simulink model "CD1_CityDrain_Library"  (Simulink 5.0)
settings: Solver=FixedStepDiscrete  StartTime=0  StopTime=36000  FixedStep=300  RelTol=1e-3
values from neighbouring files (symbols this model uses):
  table = A(2:end,1:end)    [CD1_mfun_rainread.m]    (also in CD1_sfun_rainread.m = [table; table(end,1)+tablestep -1])
  tablestep = tableEnd-tableStart    [CD1_sfun_flowread.m]
undefined symbols (not defined in the file or in its folder): Percent

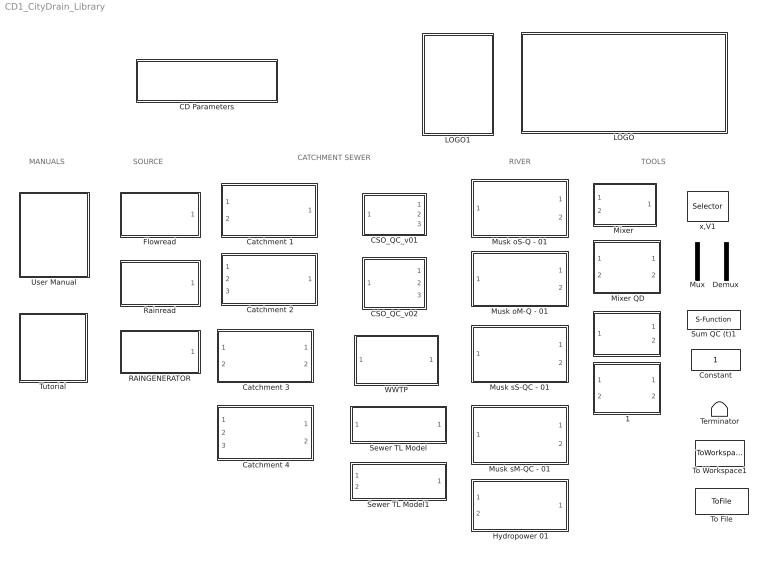
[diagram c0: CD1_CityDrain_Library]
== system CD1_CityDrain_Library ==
  note: TOOLS
  note: SOURCE
  note: RIVER
  note: CATCHMENT SEWER
  note: MANUALS
  " " : Subsystem  mask(Splitter){n_comp=1, values=40, mode=Percent [0-100]}
      mask prompts: n_comp "Number of components"; values "Fraction / Amount directed to Q1"; mode "Splitting mode"
      mask help: Splitter parameter.
      mask init:
      | % reading the toplevel systems' name 
      | % --> Plant file name;
      | tls=bdroot(gcb); 
      | % Obtaining the fixed sampling time
      | t_samp_char=get_param(tls, 'FixedStep');
      | % Convertion to numeric value
      | tstep = str2num(t_samp_char);
  " 1" : Subsystem  mask(Wrong Connect){n_comp=1, values_rain=15, mode_rain=Percent [0-100], values_dwf=23, mode_dwf=Percent [0-100]}
      mask prompts: n_comp "Number of components"; values_rain "Fraction Qr --> Qdwf"; mode_rain "Splitting mode"; values_dwf "Fraction Qdwf --> Qr"; mode_dwf "Splitting mode"
      mask help: The block simulates wrong connections given in a seperate sewer system. MAgnitudes of wrong connections are described by fraction percentages (or quanities) diverted from or to the stormwater pipe.
      mask init:
      | % reading the toplevel systems' name 
      | % --> Plant file name;
      | tls=bdroot(gcb); 
      | % Obtaining the fixed sampling time
      | t_samp_char=get_param(tls, 'FixedStep');
      | % Convertion to numeric value
      | tstep = str2num(t_samp_char);
  " Catchment 1" : Subsystem  mask(Catchment CSS - Type A){area=100, rfcoeff=0.5, initloss=1, permloss=1, n_ta=5, n_comp=1, Rain_C=[0.5], DWF_C=[1]}
      mask prompts: area "Area in [ha]"; rfcoeff "Runoff coefficient (0 - 1)"; initloss "Initial Loss in [mm]"; permloss "Permanent loss in [mm/day]"; n_ta "No of Timesteps (transport time) / No of subareas n [-]"; n_comp "No of pollutant components"; Rain_C "Vector of Rain-Conc. [g/m3]"; DWF_C "Vector of DWF-Conc. [g/m3]"
      mask help: Simple model of an urban catchment with Combined sewer system (CSS). Input ( r ) is a continuous stream of rain data in [mm/DT]. Input (dwf) is the dry weather flow in [m3/s]. Pollutants concentrations are considered as constant over time. The block contains an initial loss model for runoff generation, a time-area model for overland flow computation and a mixing model for computing runoff concentrations for n components.
      mask init:
      | % location of catchment drawing
      | x=0;
      | y=-10;
      | % reading the toplevel systems' name 
      | % --> Plant file name;
      | tls=bdroot(gcb); 
      | % Obtaining the fixed sampling time
      | t_samp_char=get_param(tls, 'FixedStep');
      | % Convertion to numeric value
      | tstep = str2num(t_samp_char); 
      | 
      | %convertion form mm/day --> mm/DT
      | permloss=permloss/86400*tstep;
      | area=area*10000;
  " Catchment 2" : Subsystem  mask(Catchment CSS - Type B){area=20, rfcoeff=0.5, initloss=1, permloss=1, n_ta=5, n_comp=1, Rain_C=[0.5]}
      mask prompts: area "Area in [ha]"; rfcoeff "Runoff coefficient (0 - 1)"; initloss "Initial Loss in [mm]"; permloss "Permanent loss in [mm/day]"; n_ta "No of Timesteps (transport time) / No of subareas n [-]"; n_comp "No of pollutant components"; Rain_C "Vector of Rain-Conc. [g/m3]"
      mask help: Simple model of an urban catchment. Input ( r ) is a continuous stream of rain data in [mm/DT]. Input (DWF) is the dry weather flow. Input (QP) is the parasite water flow entering. Pollutants concentrations for rain are considered constant over time. The block contains an initial loss model for runoff generation, a time/area model for overland flow computation and a mixing model for computing runoff concentrations for n components.
      mask init:
      | % location of catchment drawing
      | x=0;
      | y=-10;
      | % reading the toplevel systems' name 
      | % --> Plant file name;
      | tls=bdroot(gcb); 
      | % Obtaining the fixed sampling time
      | t_samp_char=get_param(tls, 'FixedStep');
      | % Convertion to numeric value
      | tstep = str2num(t_samp_char); 
      | 
      | %convertion form mm/day --> mm/DT
      | permloss=permloss/86400*tstep;
      | area=area*10000;
  " Catchment 3" : Subsystem  mask(Catchment SSS - Type A){area=20, rfcoeff=0.5, initloss=1, permloss=1, n_ta=5, n_comp=2, Rain_C=[0.5 0.2], DWF_C=[2 3]}
      mask prompts: area "Area in [ha]"; rfcoeff "Runoff coefficient (0 - 1)"; initloss "Initial Loss in [mm]"; permloss "Permanent loss in [mm/day]"; n_ta "No of Timesteps (transport time) / No of subareas n [-]"; n_comp "No of pollutant components"; Rain_C "Vector of Rain-Conc. [g/m3]"; DWF_C "Vector of DWF-Conc. [g/m3]"
      mask help: Simple model of an urban catchment with Seperate sewer system (SSS). Input ( r ) is a continuous stream of rain data in [mm/DT]. Input ( dwf ) is the dry weather flow in [m3/s]. Pollutants concentrations are considered constant over time.The block contains an initial loss model for runoff generation, a time-area model for overland flow computation and a mixing model for computing runoff concentrations for n components.
      mask init:
      | % location of catchment drawing
      | x=0;
      | y=-10;
      | % reading the toplevel systems' name 
      | % --> Plant file name;
      | tls=bdroot(gcb); 
      | % Obtaining the fixed sampling time
      | t_samp_char=get_param(tls, 'FixedStep');
      | % Convertion to numeric value
      | tstep = str2num(t_samp_char); 
      | 
      | %convertion form mm/day --> mm/DT
      | permloss=permloss/86400*tstep;
      | area=area*10000;
  " Catchment 4" : Subsystem  mask(Catchment SSS - Type B){area=20, rfcoeff=0.5, initloss=1, permloss=1, n_ta=5, n_comp=1, Rain_C=[0.5]}
      mask prompts: area "Area in [ha]"; rfcoeff "Runoff coefficient (0 - 1)"; initloss "Initial Loss in [mm]"; permloss "Permanent loss in [mm/day]"; n_ta "No of Timesteps (transport time) / No of subareas n [-]"; n_comp "No of pollutant components"; Rain_C "Vector of Rain-Conc. [g/m3]"
      mask help: Simple model of an urban catchment. Input ( r ) is a continuous stream of rain data in [mm/DT]. Input (DWF) is the dry weather flow. Input (QP) is parasite water flow entering diluting the DWF. Pollutants concentrations for stormwater Qr are considered constant over time. The block contains an initial loss model for runoff generation, a time/area model for overland flow computation and a mixing model for computing runoff concentrations for n components.
      mask init:
      | % location of catchment drawing
      | x=0;
      | y=-10;
      | % reading the toplevel systems' name 
      | % --> Plant file name;
      | tls=bdroot(gcb); 
      | % Obtaining the fixed sampling time
      | t_samp_char=get_param(tls, 'FixedStep');
      | % Convertion to numeric value
      | tstep = str2num(t_samp_char); 
      | 
      | %convertion form mm/day --> mm/DT
      | permloss=permloss/86400*tstep;
      | area=area*10000;
  " Hydropower 01" : Subsystem  mask(HYDROPOWER){n_comp=3, C_Stream=[1 2 3]}
      mask prompts: n_comp "No of components"; C_Stream "Vector of Stream-Conc. g/m3"
      mask help: Hydropower block for modelling downstream release of water. Upstream concnetration of baseflow ( qo ) and additional flow ( qa ) are considered constant. Used function: CD1_sfun_hydropower
      mask init:
      | % reading the toplevel systems' name 
      | % --> Plant file name;
      | tls=bdroot(gcb); 
      | % Obtaining the fixed sampling time
      | t_samp_char=get_param(tls, 'FixedStep');
      | % Convertion to numeric value
      | tstep = str2num(t_samp_char);
  " Mixer QD" : Subsystem  mask(Mixer QD){n_comp=3, Cmcl=[3 3 3]}
      mask prompts: n_comp "Number of pollutants [ - ]"; Cmcl "MCL - Vector of max. concentration limits [g/m3]"
      mask help: Performes mixing of pollutant fluxes Qw and Qo in accordance to their hydraulic load. Qo is considered to be the less pollluted flux. In addition the required increase of Qo is calculated for meeting required MCL (maximum concentration limits) defined by user input. Function used: CD1_sfun_mixing_QC_QD.m
      mask init:
      | % reading the toplevel systems' name 
      | % --> Plant file name;
      | tls=bdroot(gcb); 
      | % Obtaining the fixed sampling time
      | t_samp_char=get_param(tls, 'FixedStep');
      | % Convertion to numeric value
      | tstep = str2num(t_samp_char);
  CD Parameters : Subsystem  mask(City Drain 1.0 - Simulation parameters ){t_step=300, t_start=0, t_stop=36000}
      mask prompts: t_step "Sampling Time [s]"; t_start "Start Time [s]"; t_stop "Stop Time [s]"
      mask help: Block that sets the global parameters required in City Drain 1.0. Following paramters are set without user's input: - 'Solver' --> 'FixedStepDiscrete' - 'TimeSaveName' --> 'cd_time' - 'Decimation' --> '1' - 'LimitDataPoints' --> 'off'
      mask init:
      | % toplevel systems' name --> Plant file name;
      | tls=bdroot(gcb); 
      | set_param(tls, 'Solver', 'FixedStepDiscrete'); 
      | set_param(tls, 'TimeSaveName', 'cd_time');
      | set_param(tls, 'Decimation', '1');
      | set_param(tls, 'LimitDataPoints', 'off');
      | set_param(tls, 'ScreenColor', 'white');
      | 
      | tstep_char=num2str(t_step); % Setting the discrete time step
      | set_param(tls, 'FixedStep', tstep_char); 
      | 
      | tstart_char=num2str(t_start); % Setting the start time
      | set_param(tls, 'StartTime', tstart_char); 
      | 
      | tstop_char=num2str(t_stop); % Setting the stop time
      | set_param(tls, 'StopTime', tstop_char);
  CSO_QC_v01 : Subsystem  mask(CSO Typ A - Combined sewer overflow){Vmax=300, Qemax=0.1, n_comp=2}
      mask prompts: Vmax "Basin Volume [m3]"; Qemax "Maximum Effluent flow [m3/s]"; n_comp "Number of Pollutants [-]"
      mask help: Combined sewer overflow structure. Diverts the inflow given into effluent and overflow. The model implemented consideres hydraulics and pollutant routing by full mixing in the structure. Function used: CD1_sfun_cso_A.m
      mask init:
      | % reading the toplevel systems' name 
      | % --> Plant file name;
      | tls=bdroot(gcb); 
      | % Obtaining the fixed sampling time
      | t_samp_char=get_param(tls, 'FixedStep');
      | % Convertion to numeric value
      | tstep = str2num(t_samp_char);
  CSO_QC_v02 : Subsystem  mask(CSO Typ B - Combined sewer overflow){Vmax=300, Qemax=0.1, n_comp=1, n_sed=[0.2]}
      mask prompts: Vmax "Basin Volume (m3)"; Qemax "Maximum Effluent flow [m3/s]"; n_comp "Number of Pollutants [-]"; n_sed "n-sed (Vect. of Sed. Coefficients)"
      mask help: Combined sewer overflow structure. Diverts the inflow given into effluent and overflow. The model implemented consideres hydraulics and pollutant routing by full mixing in the structure. In addition to Type A a retenetion/sedimentation factor is introduced. The factor may be used for applying different ratios in pollutant concentration for effluent flow (QE) and overflow (QW). Function used: CD1_sfun_cso_B.m
      mask init:
      | % reading the toplevel systems' name 
      | % --> Plant file name;
      | tls=bdroot(gcb); 
      | % Obtaining the fixed sampling time
      | t_samp_char=get_param(tls, 'FixedStep');
      | % Convertion to numeric value
      | tstep = str2num(t_samp_char);
  Constant : Constant
  Demux : Demux  Outputs=[13,1]
  Flowread : Subsystem  mask(CD1_Flowread){table0='Input_CSO_QC_Test_01.txt', dtype=Composite sample, crep=off}
      mask prompts: table0 "Filename"; dtype "Data type"; crep "Cylic repitition"
      mask help: Reads flowdata (Q) and substance concentration (Ci) associated from ascii file. Used function: CD1_sfun_flowread.m CD1_mfun_flowread.m
      mask init:
      | table=CD1_mfun_flowread(table0);
      | 
      | 
      | % reading the toplevel systems' name 
      | % --> Plant file name;
      | tls=bdroot(gcb); 
      | % Obtaining the fixed sampling time
      | t_samp_char=get_param(tls, 'FixedStep');
      | % Convertion to numeric value
      | tstep = str2num(t_samp_char);
  LOGO : Subsystem
  LOGO1 : Subsystem
  "Mixer " : Subsystem  mask(Mixer){n_comp=1}
      mask prompts: n_comp "Number of pollutants [ - ]"
      mask help: Performes mixing of pollutant fluxes Q1 and Q2 in accordance to their hydraulic load. Function used: CD1_sfun_mixing_QC.m
      mask init:
      | % reading the toplevel systems' name 
      | % --> Plant file name;
      | tls=bdroot(gcb); 
      | % Obtaining the fixed sampling time
      | t_samp_char=get_param(tls, 'FixedStep');
      | % Convertion to numeric value
      | tstep = str2num(t_samp_char);
  Musk oM-Q - 01 : Subsystem  mask(Muskingum - Cunge flood rooting (original scheme)){K=900, X=0.2, N=2}
      mask prompts: K "K (travel time of one subreach) [ s ]"; X "X (weighing factor) [ - ]"; N "N (Number of sub-reaches) [ - ]"
      mask help: Flood routing using the original scheme by Muskingum-Cunge for multiple river stretches for hydraulic routing only. The block accepts flow inputs and returns effluent fluxes and current stated of retained volume. Intial Conditions: V=0; and Qe=0; Function used: CD1_sfun_Muskingum_oM_Q.m
      mask init:
      | m=[5,5];%Offset for arrow 
      | l=[65,15];%Offset for arrow 
      | x=0; 
      | y=-15; %Offset for river
      | 
      | % reading the toplevel systems' name-> Plant file name;
      | tls=bdroot(gcb); 
      | % Obtaining the fixed sampling time
      | tstep_char=get_param(tls, 'FixedStep');
      | % Convertion to numeric value
      | dt = str2num(tstep_char); 
      | 
      | 
      | 
      | %Muskingum parameters
      | D=K.*(1-X)+0.5.*dt;
      | C0=(0.5.*dt-K.*X)./D;
      | C1=(0.5.*dt+K.*X)./D;
      | C2=(K.*(1-X)-0.5.*dt)./D;
  Musk oS-Q - 01 : Subsystem  mask(Muskingum - Cunge flood rooting (original scheme)){K=300, X=0.2}
      mask prompts: K "K (travel time of the reach) [s]"; X "X (weighing factor)  [ - ]"
      mask help: Flood routing unsing the original scheme by Muskingum-Cunge for a single river stretch for hydraulic routing only. The block accepts flow inputs and returns effluent fluxes and current stated of retained volume. Intial Conditions: V=0; and Qe=0; Function used: CD1_sfun_Muskingum_oS_Q.m
      mask init:
      | % reading the toplevel systems' name 
      | % --> Plant file name;
      | tls=bdroot(gcb); 
      | % Obtaining the fixed sampling time
      | t_samp_char=get_param(tls, 'FixedStep');
      | % Convertion to numeric value
      | dt = str2num(t_samp_char); 
      | 
      | %Muskingum parameters
      | D=K.*(1-X)+0.5.*dt;
      | C0=(0.5.*dt-K.*X)./D;
      | C1=(0.5.*dt+K.*X)./D;
      | C2=(K.*(1-X)-0.5.*dt)./D;
  Musk sM-QC - 01 : Subsystem  mask(Muskingum - Cunge flood rooting - simplified scheme){K=300, X=0.3, n_comp=1, N=1}
      mask prompts: K "K (travel time of a subreach) [s]"; X "X (weighing factor)  [ - ]"; n_comp "Number of pollutants [ - ]"; N "N (Number of sub-reaches) [ - ]"
      mask help: Flood routing using the Muskingum-Cunge scheme for multiple river stretches for hydraulic and pollutant routing. The block accepts flow inputs and returns effluent fluxes and current stated of retained volume. Intial Conditions: V=0; and Qe=0; Function used: CD1_sfun_Muskingum_sM_QC.m
      mask init:
      | m=[5,5];%Offset for arrow 
      | l=[65,15];%Offset for arrow 
      | x=0; 
      | y=-15; %Offset for river
      | 
      | % reading the toplevel systems' name 
      | % --> Plant file name;
      | tls=bdroot(gcb); 
      | % Obtaining the fixed sampling time
      | t_samp_char=get_param(tls, 'FixedStep');
      | % Convertion to numeric value
      | dt = str2num(t_samp_char); 
      | 
      | %Muskingum parameters
      | CA=0.5.*dt-K.*X;
      | CB=0.5.*dt+K.*(1-X);
  Musk sS-QC - 01 : Subsystem  mask(Muskingum - Cunge flood rooting ){K=300, X=0.2, n_comp=1}
      mask prompts: K "K (travel time of the reach) [s]"; X "X (weighing factor)  [ - ]"; n_comp "Number of pollutants n [ - ]"
      mask help: Flood routing using the Muskingum-Cunge scheme for a single river stretch. Routing is provide for hydraulics and pollutants using a simplified discrete scheme. The block accepts flow inputs and returns effluent fluxes and current states of retained volume. Intial Conditions: V=0; and Qe=0; Function used: CD1_sfun_Muskingum_sS_QC.m
      mask init:
      | % reading the toplevel systems' name 
      | % --> Plant file name;
      | tls=bdroot(gcb); 
      | % Obtaining the fixed sampling time
      | t_samp_char=get_param(tls, 'FixedStep');
      | % Convertion to numeric value
      | dt = str2num(t_samp_char); 
      | 
      | %Muskingum parameters
      | CA=0.5.*dt-K.*X;
      | CB=0.5.*dt+K.*(1-X);
  Mux : Mux  Inputs=[13,1]
  RAINGENERATOR : Subsystem  mask(Rain Generator){param=[1,3,0.2,0.3]}
      mask prompts: param "Parameters [a,b,c,d]"
      mask help: Generates rain pattern by means of stochstics.
      mask init:
      | a=param(1);
      | b=param(2);
      | c=param(3);
      | d=param(4);
      | 
      | % reading the toplevel systems' name 
      | % --> Plant file name;
      | tls=bdroot(gcb); 
      | % Obtaining the fixed sampling time
      | t_samp_char=get_param(tls, 'FixedStep');
      | % Convertion to numeric value
      | t_step = str2num(t_samp_char);
  Rainread : Subsystem  mask(Rain Read){table0='test2.km2', crep=off}
      mask prompts: table0 "Filename"; crep "Cylic repitition"
      mask help: Read raindata from ASCII File in following formats: *.ixx ... Format used by the Austrian Hydrographic Service. *.km2 ... Format used in the Mouse Software from DHI (Danish Hydraulic Institute) *.mse ... modified mse format used in Mouse Software from DHI (Danish Hydraulic Institute) Used function: CD1_mfun_rainread.m
      mask init:
      | % cache table size set to 1000
      | %table=zeros(1000,2)
      | [table,tablestep]=CD1_mfun_rainread(table0);
      | 
      | % reading the toplevel systems' name 
      | % --> Plant file name;
      | tls=bdroot(gcb); 
      | % Obtaining the fixed sampling time
      | t_samp_char=get_param(tls, 'FixedStep');
      | % Convertion to numeric value
      | tstep = str2num(t_samp_char);
  Sewer TL Model : Subsystem  mask(SEWER Translation Model){n_elem=5, n_comp=1}
      mask prompts: n_elem "Transport time in No of Timesteps ()"; n_comp "Number of Components ()"
      mask help: Block accepts Qi as inflow carrying a number of pollutants (n_comp) Output is the flow at the end of sewer Qe Function used: CD1_sfun_sewer_tlmodel.m
      mask init:
      | %arrow location in icon
      | kx=70;
      | ky=25;
      | % picture location
      | x=20;y=25;
      | 
      | 
      | % reading the toplevel systems' name 
      | % --> Plant file name;
      | tls=bdroot(gcb); 
      | % Obtaining the fixed sampling time
      | t_samp_char=get_param(tls, 'FixedStep');
      | % Convertion to numeric value
      | tstep = str2num(t_samp_char);
  Sewer TL Model1 : Subsystem  mask(SEWER TL - Translation Model){n_elem=5, n_comp=1}
      mask prompts: n_elem "Transport time in No of Timesteps ()"; n_comp "Number of Components ()"
      mask help: Block accepts Qi as inflow carrying a number of pollutants (n_comp). Flow of parasite water (Qp) is optional. Output is the flow at the end of sewer Qe. Function used: CD1_sfun_sewer_tlmodel.m
      mask init:
      | %arrow location in icon
      | kx=70;
      | ky=25;
      | % picture location
      | x=20;y=25;
      | 
      | 
      | % reading the toplevel systems' name 
      | % --> Plant file name;
      | tls=bdroot(gcb); 
      | % Obtaining the fixed sampling time
      | t_samp_char=get_param(tls, 'FixedStep');
      | % Convertion to numeric value
      | tstep = str2num(t_samp_char);
  Sum QC (t)1 : S-Function  FunctionName=CD1_sfun_sum_QC  Parameters=n_p, tstep  mask(Cumulation of Masses){n_p=1}
      mask prompts: n_p "Number of pollutants [ - ]"
      mask help: This block returns the total hydraulic load V [m3] and the pollutant load M [g] during the simulation run. Function used: CD1_sfun_sum_QC_t.m
      mask init:
      | % reading the toplevel systems' name 
      | % --> Plant file name;
      | tls=bdroot(gcb); 
      | % Obtaining the fixed sampling time
      | t_samp_char=get_param(tls, 'FixedStep');
      | % Convertion to numeric value
      | tstep = str2num(t_samp_char);
  Terminator : Terminator
  To File : ToFile  Filename=output.mat
  To Workspace1 : ToWorkspace  VariableName=yout  SampleTime=-1  SaveFormat=Array
  Tutorial : Subsystem
  User Manual : Subsystem
  WWTP : Subsystem  mask(WWTP){REmin=[0.85 0.8 0.75], Cemax=[5 .2 .5], n_comp=3}
      mask prompts: REmin "Removal Efficiency REmin [-]"; Cemax "Maximum effluent concnetration Cemax [g/m³]"; n_comp "Number of Components ()"
      mask help: Simple WWTP model. Inflow given is treated according to userdefined maximum concnetration limits and treatment efficiencies. Function used: CD1_sfun_WWTP.m
      mask init:
      | % reading the toplevel systems' name 
      | % --> Plant file name;
      | tls=bdroot(gcb); 
      | % Obtaining the fixed sampling time
      | t_samp_char=get_param(tls, 'FixedStep');
      | % Convertion to numeric value
      | tstep = str2num(t_samp_char); 
      | 
      | RE=REmin;
      | for i=1:n_comp
      | 	if REmin(i) < 0 
      | 		RE(i)=0;
      | 		fprintf('WARNING, Block WWTP:  Removal efficientc of component %u has set to 0, User input REmin <0 \n',i);
      | 	elseif REmin(i) > 1
      | 		RE(i)=1;
      | 		fprintf('WARNING, Block WWTP:  Removal efficientc of component %u has set to 1, User input REmin >1 \n',i);
      | 	else
      | 		RE(i)=REmin(i);
      | 	end
      | end
      | fprintf('\n');
  x,V1 : Selector  Elements=(1:14)  InputPortWidth=3*14

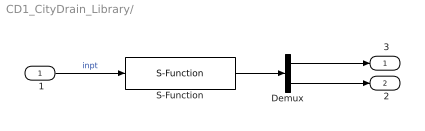
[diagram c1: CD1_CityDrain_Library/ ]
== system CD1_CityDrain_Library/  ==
  " 1" : Inport
  Demux : Demux  Outputs=2
  S-Function : S-Function  FunctionName=CD1_sfun_splitter  Parameters=n_comp,values,mode,tstep
  " 3" : Outport
  " 2" : Outport  Port=2
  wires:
  " 1"/1 -> S-Function/1  "inpt"
  S-Function/1 -> Demux/1
  Demux/1 -> " 3"/1
  Demux/2 -> " 2"/1

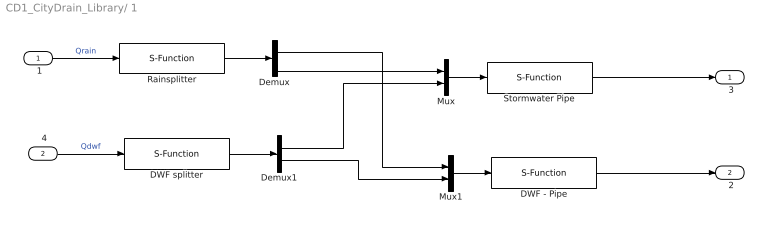
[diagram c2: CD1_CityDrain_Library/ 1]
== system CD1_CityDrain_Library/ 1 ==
  " 1" : Inport
  " 4" : Inport  Port=2
  DWF - Pipe : S-Function  FunctionName=CD1_sfun_mixing_QC  Parameters=n_comp,tstep
  DWF splitter : S-Function  FunctionName=CD1_sfun_splitter  Parameters=n_comp,values_dwf,mode_dwf,tstep
  Demux : Demux  Outputs=2
  Demux1 : Demux  Outputs=2
  Mux : Mux  Inputs=2
  Mux1 : Mux  Inputs=2
  Rainsplitter : S-Function  FunctionName=CD1_sfun_splitter  Parameters=n_comp,values_rain,mode_rain,tstep
  Stormwater Pipe : S-Function  FunctionName=CD1_sfun_mixing_QC  Parameters=n_comp,tstep
  " 3" : Outport
  " 2" : Outport  Port=2
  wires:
  " 1"/1 -> Rainsplitter/1  "Qrain"
  Rainsplitter/1 -> Demux/1
  " 4"/1 -> DWF splitter/1  "Qdwf"
  DWF splitter/1 -> Demux1/1
  Mux/1 -> Stormwater Pipe/1
  Demux/2 -> Mux/1
  Demux1/1 -> Mux/2
  Mux1/1 -> DWF - Pipe/1
  Demux/1 -> Mux1/1
  Demux1/2 -> Mux1/2
  DWF - Pipe/1 -> " 2"/1
  Stormwater Pipe/1 -> " 3"/1

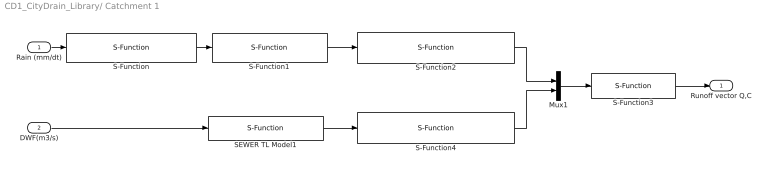
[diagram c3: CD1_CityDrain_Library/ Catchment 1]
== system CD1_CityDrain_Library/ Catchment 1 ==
  Rain (mm/dt) : Inport
  DWF(m3/s) : Inport  Port=2
  Mux1 : Mux  Inputs=[n_comp+1,n_comp+1]
  S-Function : S-Function  FunctionName=CD1_sfun_catchment_lossmodel  Parameters=initloss,permloss,rfcoeff
  S-Function1 : S-Function  FunctionName=CD1_sfun_catchment_tamodel  Parameters=n_ta
  S-Function2 : S-Function  FunctionName=CD1_sfun_catchment_flowmodel_SW  Parameters=area,n_comp,Rain_C,tstep
  S-Function3 : S-Function  FunctionName=CD1_sfun_mixing_QC  Parameters=n_comp,tstep
  S-Function4 : S-Function  FunctionName=CD1_sfun_catchment_flowmodel_DWF  Parameters=n_comp,DWF_C,tstep
  SEWER TL Model1 : S-Function  FunctionName=CD1_sfun_sewer_tlmodel  Parameters=n_ta,0,tstep
  Runoff vector Q,C : Outport
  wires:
  S-Function/1 -> S-Function1/1
  Rain (mm/dt)/1 -> S-Function/1
  DWF(m3/s)/1 -> SEWER TL Model1/1
  Mux1/1 -> S-Function3/1
  S-Function3/1 -> Runoff vector Q,C/1
  S-Function1/1 -> S-Function2/1
  SEWER TL Model1/1 -> S-Function4/1
  S-Function2/1 -> Mux1/1
  S-Function4/1 -> Mux1/2

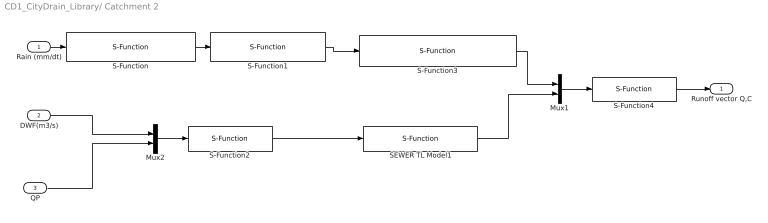
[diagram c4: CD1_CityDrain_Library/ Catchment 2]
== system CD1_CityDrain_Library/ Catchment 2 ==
  Rain (mm/dt) : Inport
  DWF(m3/s) : Inport  Port=2
  QP : Inport  Port=3
  Mux1 : Mux  Inputs=[n_comp+1,n_comp+1]
  Mux2 : Mux  Inputs=[n_comp+1,n_comp+1]
  S-Function : S-Function  FunctionName=CD1_sfun_catchment_lossmodel  Parameters=initloss,permloss,rfcoeff
  S-Function1 : S-Function  FunctionName=CD1_sfun_catchment_tamodel  Parameters=n_ta
  S-Function2 : S-Function  FunctionName=CD1_sfun_mixing_QC  Parameters=n_comp,tstep
  S-Function3 : S-Function  FunctionName=CD1_sfun_catchment_flowmodel_SW  Parameters=area,n_comp,Rain_C,tstep
  S-Function4 : S-Function  FunctionName=CD1_sfun_mixing_QC  Parameters=n_comp,tstep
  SEWER TL Model1 : S-Function  FunctionName=CD1_sfun_sewer_tlmodel  Parameters=n_ta,n_comp,tstep
  Runoff vector Q,C : Outport
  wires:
  S-Function/1 -> S-Function1/1
  Rain (mm/dt)/1 -> S-Function/1
  Mux1/1 -> S-Function4/1
  S-Function4/1 -> Runoff vector Q,C/1
  S-Function3/1 -> Mux1/1
  S-Function1/1 -> S-Function3/1
  Mux2/1 -> S-Function2/1
  S-Function2/1 -> SEWER TL Model1/1
  DWF(m3/s)/1 -> Mux2/1
  QP/1 -> Mux2/2
  SEWER TL Model1/1 -> Mux1/2

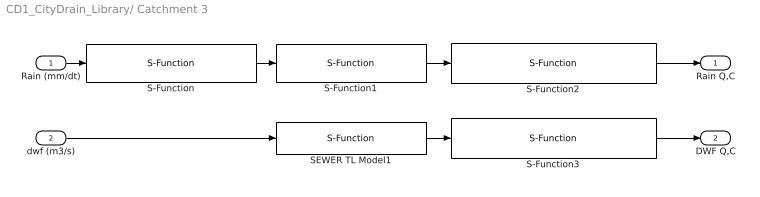
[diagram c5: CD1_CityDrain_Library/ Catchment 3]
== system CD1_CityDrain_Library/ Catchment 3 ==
  Rain (mm/dt) : Inport
  dwf (m3/s) : Inport  Port=2
  S-Function : S-Function  FunctionName=CD1_sfun_catchment_lossmodel  Parameters=initloss,permloss,rfcoeff
  S-Function1 : S-Function  FunctionName=CD1_sfun_catchment_tamodel  Parameters=n_ta
  S-Function2 : S-Function  FunctionName=CD1_sfun_catchment_flowmodel_SW  Parameters=area,n_comp,Rain_C,tstep
  S-Function3 : S-Function  FunctionName=CD1_sfun_catchment_flowmodel_DWF  Parameters=n_comp,DWF_C,tstep
  SEWER TL Model1 : S-Function  FunctionName=CD1_sfun_sewer_tlmodel  Parameters=n_ta,0,tstep
  Rain Q,C : Outport
  DWF Q,C : Outport  Port=2
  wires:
  S-Function2/1 -> Rain Q,C/1
  S-Function/1 -> S-Function1/1
  Rain (mm/dt)/1 -> S-Function/1
  dwf (m3/s)/1 -> SEWER TL Model1/1
  S-Function1/1 -> S-Function2/1
  SEWER TL Model1/1 -> S-Function3/1
  S-Function3/1 -> DWF Q,C/1

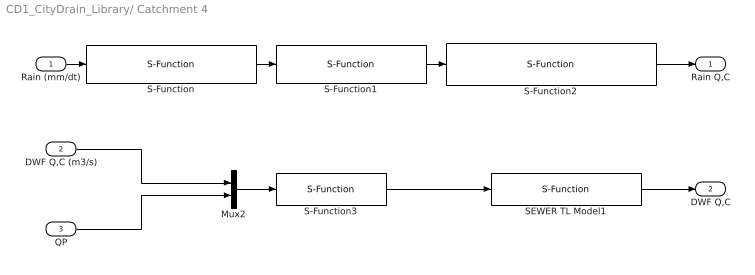
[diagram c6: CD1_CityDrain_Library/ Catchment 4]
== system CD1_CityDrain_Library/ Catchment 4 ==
  Rain (mm/dt) : Inport
  DWF Q,C (m3/s) : Inport  Port=2
  QP : Inport  Port=3
  Mux2 : Mux  Inputs=[n_comp+1,n_comp+1]
  S-Function : S-Function  FunctionName=CD1_sfun_catchment_lossmodel  Parameters=initloss,permloss,rfcoeff
  S-Function1 : S-Function  FunctionName=CD1_sfun_catchment_tamodel  Parameters=n_ta
  S-Function2 : S-Function  FunctionName=CD1_sfun_catchment_flowmodel_SW  Parameters=area,n_comp,Rain_C,tstep
  S-Function3 : S-Function  FunctionName=CD1_sfun_mixing_QC  Parameters=n_comp,tstep
  SEWER TL Model1 : S-Function  FunctionName=CD1_sfun_sewer_tlmodel  Parameters=n_ta,n_comp,tstep
  Rain Q,C : Outport
  DWF Q,C : Outport  Port=2
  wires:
  S-Function2/1 -> Rain Q,C/1
  S-Function/1 -> S-Function1/1
  Rain (mm/dt)/1 -> S-Function/1
  S-Function1/1 -> S-Function2/1
  SEWER TL Model1/1 -> DWF Q,C/1
  Mux2/1 -> S-Function3/1
  S-Function3/1 -> SEWER TL Model1/1
  DWF Q,C (m3/s)/1 -> Mux2/1
  QP/1 -> Mux2/2

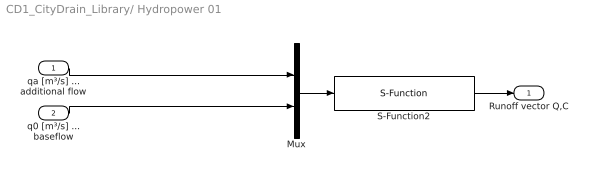
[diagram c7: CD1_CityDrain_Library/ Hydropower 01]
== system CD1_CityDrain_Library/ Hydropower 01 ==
  qa [m³/s] ... additional flow : Inport
  q0 [m³/s] ... baseflow : Inport  Port=2
  Mux : Mux  Inputs=2
  S-Function2 : S-Function  FunctionName=CD1_sfun_hydropower  Parameters=n_comp,C_Stream,tstep
  Runoff vector Q,C : Outport
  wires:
  Mux/1 -> S-Function2/1
  S-Function2/1 -> Runoff vector Q,C/1
  q0 [m³/s] ... baseflow/1 -> Mux/2
  qa [m³/s] ... additional flow/1 -> Mux/1

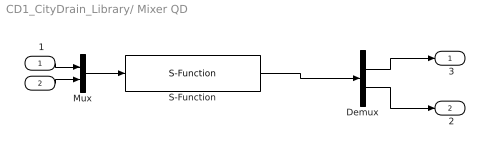
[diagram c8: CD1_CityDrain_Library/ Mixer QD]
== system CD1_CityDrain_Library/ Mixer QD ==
  " 1" : Inport
  " " : Inport  Port=2
  Demux : Demux  Outputs=[ (n_comp+1) (n_comp+1)]
  Mux : Mux  Inputs=2
  S-Function : S-Function  FunctionName=CD1_sfun_mixing_QC_QD  Parameters=n_comp,tstep,Cmcl
  " 3" : Outport
  " 2" : Outport  Port=2
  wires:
  " "/1 -> Mux/2
  " 1"/1 -> Mux/1
  Mux/1 -> S-Function/1
  Demux/1 -> " 3"/1
  Demux/2 -> " 2"/1
  S-Function/1 -> Demux/1

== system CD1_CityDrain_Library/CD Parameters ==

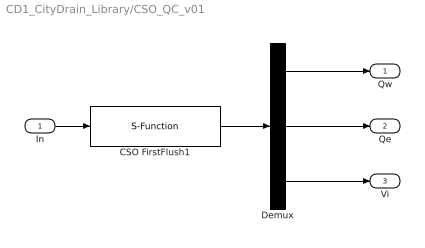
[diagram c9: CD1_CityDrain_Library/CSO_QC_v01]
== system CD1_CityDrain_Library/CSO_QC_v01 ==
  In : Inport
  CSO FirstFlush1 : S-Function  FunctionName=CD1_sfun_cso_A  Parameters=Vmax,Qemax,n_comp,tstep
  Demux : Demux  Outputs=[ (n_comp+1) (n_comp+1) (n_comp+1)]
  Qw : Outport
  Qe : Outport  Port=2
  Vi : Outport  Port=3
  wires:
  In/1 -> CSO FirstFlush1/1
  CSO FirstFlush1/1 -> Demux/1
  Demux/1 -> Qw/1
  Demux/2 -> Qe/1
  Demux/3 -> Vi/1

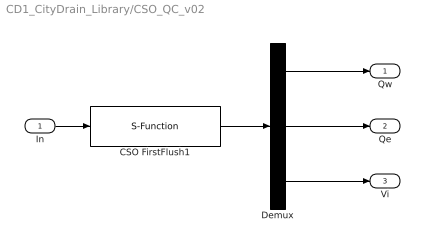
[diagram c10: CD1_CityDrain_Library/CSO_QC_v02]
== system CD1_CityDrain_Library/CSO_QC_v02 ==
  In : Inport
  CSO FirstFlush1 : S-Function  FunctionName=CD1_sfun_cso_B  Parameters=Vmax,Qemax,n_comp,n_sed,tstep
  Demux : Demux  Outputs=[ (n_comp+1) (n_comp+1) (n_comp+1)]
  Qw : Outport
  Qe : Outport  Port=2
  Vi : Outport  Port=3
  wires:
  In/1 -> CSO FirstFlush1/1
  CSO FirstFlush1/1 -> Demux/1
  Demux/1 -> Qw/1
  Demux/2 -> Qe/1
  Demux/3 -> Vi/1

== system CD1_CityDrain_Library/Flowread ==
  flowread : S-Function  FunctionName=CD1_sfun_flowread  Parameters=dtype,crep,table,tstep
  out_1 : Outport
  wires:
  flowread/1 -> out_1/1

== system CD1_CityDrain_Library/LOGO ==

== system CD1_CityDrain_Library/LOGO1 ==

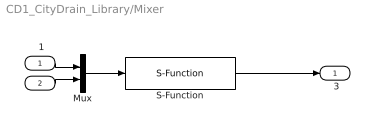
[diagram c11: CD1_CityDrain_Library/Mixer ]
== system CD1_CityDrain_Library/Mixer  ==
  " 1" : Inport
  " " : Inport  Port=2
  Mux : Mux  Inputs=[n_comp+1,n_comp+1]
  S-Function : S-Function  FunctionName=CD1_sfun_mixing_QC  Parameters=n_comp,tstep
  " 3" : Outport
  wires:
  " "/1 -> Mux/2
  S-Function/1 -> " 3"/1
  " 1"/1 -> Mux/1
  Mux/1 -> S-Function/1

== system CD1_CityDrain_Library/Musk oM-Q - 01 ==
  Qi : Inport
  Demux : Demux  Outputs=[N+1,N]
  S-Function1 : S-Function  FunctionName=CD1_sfun_Muskingum_oM_Q  Parameters=dt,N,K,X,C0,C1,C2
  Q : Outport
  V : Outport  Port=2
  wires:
  Qi/1 -> S-Function1/1
  Demux/2 -> V/1
  Demux/1 -> Q/1
  S-Function1/1 -> Demux/1

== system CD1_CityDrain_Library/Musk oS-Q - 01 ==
  Qi : Inport
  Demux : Demux  Outputs=2
  S-Function1 : S-Function  FunctionName=CD1_sfun_Muskingum_oS_Q  Parameters=dt, K, X, C0, C1, C2
  Qe : Outport
  V : Outport  Port=2
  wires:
  S-Function1/1 -> Demux/1
  Demux/1 -> Qe/1
  Demux/2 -> V/1
  Qi/1 -> S-Function1/1

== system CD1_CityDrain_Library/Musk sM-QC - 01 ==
  Qi : Inport
  Demux : Demux  Outputs=2
  S-Function1 : S-Function  FunctionName=CD1_sfun_Muskingum_sM_QC  Parameters=dt, K, X, CA, CB, n_comp,N
  Qe : Outport
  V : Outport  Port=2
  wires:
  S-Function1/1 -> Demux/1
  Demux/1 -> Qe/1
  Demux/2 -> V/1
  Qi/1 -> S-Function1/1

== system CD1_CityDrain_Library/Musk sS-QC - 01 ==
  Qi : Inport
  Demux : Demux  Outputs=2
  S-Function1 : S-Function  FunctionName=CD1_sfun_Muskingum_sS_QC  Parameters=dt, K, X, CA, CB, n_comp
  Qe : Outport
  V : Outport  Port=2
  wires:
  S-Function1/1 -> Demux/1
  Demux/1 -> Qe/1
  Demux/2 -> V/1
  Qi/1 -> S-Function1/1

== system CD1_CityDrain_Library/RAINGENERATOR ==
  S-Function : S-Function  FunctionName=CD1_sfun_raingenerator  Parameters=t_step,a,b,c,d
  Output Signal: mm/timestep : Outport
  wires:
  S-Function/1 -> Output Signal: mm/timestep/1

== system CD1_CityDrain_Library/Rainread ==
  rainread : S-Function  FunctionName=CD1_sfun_rainread  Parameters=crep,table,tablestep,tstep
  out_1 : Outport
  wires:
  rainread/1 -> out_1/1

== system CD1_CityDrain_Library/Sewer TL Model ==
  Qi : Inport
  SEWER TL Model1 : S-Function  FunctionName=CD1_sfun_sewer_tlmodel  Parameters=n_elem,n_comp,tstep
  Qe : Outport
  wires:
  Qi/1 -> SEWER TL Model1/1
  SEWER TL Model1/1 -> Qe/1

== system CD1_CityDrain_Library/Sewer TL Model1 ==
  Qi : Inport
  qp : Inport  Port=2
  Parasite water : Subsystem
  SEWER TL Model1 : S-Function  FunctionName=CD1_sfun_sewer_tlmodel  Parameters=n_elem,n_comp,tstep
  Qe : Outport
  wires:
  SEWER TL Model1/1 -> Qe/1
  Qi/1 -> Parasite water/1(Qi)
  qp/1 -> Parasite water/2(Qp)
  Parasite water/1(Oi+Qp) -> SEWER TL Model1/1

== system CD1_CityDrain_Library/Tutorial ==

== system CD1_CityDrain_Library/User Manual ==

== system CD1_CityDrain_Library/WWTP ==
  In : Inport
  WWTP v01 - 1 : S-Function  FunctionName=CD1_sfun_WWTP  Parameters=n_comp,RE,Cemax,tstep
  Qw : Outport
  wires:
  In/1 -> WWTP v01 - 1/1
  WWTP v01 - 1/1 -> Qw/1

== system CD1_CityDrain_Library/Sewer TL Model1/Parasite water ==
  Qi : Inport
  Qp : Inport  Port=2
  Mux : Mux  Inputs=[n_comp+1,n_comp+1]
  S-Function : S-Function  FunctionName=CD1_sfun_mixing_QC  Parameters=n_comp,tstep
  Oi+Qp : Outport
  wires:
  Mux/1 -> S-Function/1
  S-Function/1 -> Oi+Qp/1
  Qi/1 -> Mux/1
  Qp/1 -> Mux/2
